| Integrated Devices Technolgy, Inc.
| IBIS Model Of 82P2816
| BB_416
[IBIS ver]	3.2
[File name]	82p2816.ibs
[File Rev]	1.0
[Date]		Aug. 15, 2005
[Source]	Integrated Devices Technolgy, Inc.
[Notes]   1. Temperatures: typ=25C, min=90C, max=-40C .
   2. simulator: hspice
   3. The IBIS models are validated with hspice models
[Disclaimer]	 Integrated Device Technology, Inc. ("IDT") hereby grants
		 the user of this IBIS model a non-exclusive, nontransferable
		 license to use this IBIS model under the following terms.
		 The user is granted this license only to use the IBIS model
		 and is not granted rights to sell, copy (except as needed to
		 run the IBIS model), rent, lease or sub-license the IBIS model
		 in whole or in part, or in modified form to anyone. The User
		 may modify the IBIS model to suit its specific applications,
		 but rights to derivative works and such modifications shall
		 belong to IDT. This IBIS model is provided on an AS IS" basis
		 and IDT makes absolutely no warranty with respect to the
		 information contained herein. IDT DISCLAIMS AND CUSTOMER WAIVES
		 ALL WARRANTIES, EXPRESS AND IMPLIED, INCLUDING WARRANTIES
		 OF MERCHANTABILITY AND FITNESS FOR A PARTICULAR PURPOSE. THE
		 ENTIRE RISK AS TO QUALITY AND PERFORMANCE IS WITH THE USER ACCORDINGLY,
		 IN NO EVENT SHALL IDT BE LIABLE FOR ANY DIRECT OR
		 INDIRECT DAMAGES, WHETHER IN CONTRACT OR TORT, INCLUDING ANY
		 LOST PROFITS OR OTHER INCIDENTAL, CONSEQUENTIAL, EXEMPLARY, OR
		 PUNITIVE DAMAGES ARISING OUT OF THE USE OR APPLICATION OF THE
		 IBIS model. Further, IDT reserves the right to make changes
		 without notice to
[Copyright]	Copyright 2005, Integrated Devices Technolgy, Inc.,
   All Rights Reserved.
|   Component 82P2816
[Component]	82P2816
[Manufacturer]	Integrated Devices Technolgy, Inc.
[Package]
| variable   typ   min   max
R_pkg   0.32   0.20   0.57
L_pkg   6.21nH   3.81nH   11.4nH
C_pkg   0.91pF   0.37pF   2.25pF
[Pin]  signal_name   model_name   R_pin   L_pin   C_pin
AE16   A0   PITSN   0.40   7.41nH   0.70pF
AF16   A1   PITSN   0.37   7.24nH   0.37pF
AE13   A10   PITSN   0.27   4.86nH   0.56pF
AD15   A2   PITSN   0.26   4.33nH   0.64pF
AE15   A3   PITSN   0.33   6.06nH   0.49pF
AF15   A4   PITSN   0.33   5.99nH   0.58pF
AC14   A5   PITSN   0.25   4.16nH   0.63pF
AD14   A6   PITSN   0.30   4.76nH   0.64pF
AE14   A7   PITSN   0.31   5.65nH   0.58pF
AF14   A8   PITSN   0.34   5.72nH   0.72pF
AD13   A9   PITSN   0.30   5.24nH   0.59pF
AD17   ALE_AS   PITSN   0.34   5.34nH   0.60pF
AE20   CLKA   PITSN   0.38   7.14nH   0.65pF
AF20   CLKB   PITSN   0.41   7.05nH   0.83pF
AD20   CLKE1   PTT04   0.38   6.28nH   1.00pF
AC21   CLKT1   PTT04   0.35   5.62nH   1.33pF
AD18   CSB   PITSN   0.30   5.34nH   0.64pF
AF13   D0   PBRT16N   0.36   6.83nH   0.59pF
AC12   D1   PBRT16N   0.26   3.95nH   0.69pF
AD12   D2   PBRT16N   0.30   5.18nH   0.69pF
AE12   D3   PBRT16N   0.35   5.72nH   0.75pF
AF12   D4   PBRT16N   0.37   6.72nH   0.56pF
AD11   D5   PBRT16N   0.29   5.28nH   0.81pF
AE11   D6   PBRT16N   0.34   6.09nH   0.63pF
AF11   D7   PBRT16N   0.36   6.25nH   0.80pF
AD9   GPIO0   PBRT04N   0.32   6.20nH   0.71pF
AC8   GPIO1   PBRT04N   0.43   8.75nH   0.82pF
AC17   IM   PITSU   0.45   7.78nH   0.67pF
AD16   INT_MOTB   PITSU   0.29   5.28nH   0.51pF
AF18   INTB   PTT12   0.42   7.96nH   0.48pF
AD19   LLOS   PTT04   0.50   10.21nH   0.77pF
AC19   LLOS0   PTT04   0.45   9.39nH   1.11pF
AE21   MCKSEL0   PITSN   0.40   7.45nH   0.54pF
AD21   MCKSEL1   PITSN   0.41   7.14nH   1.10pF
AD22   MCKSEL2   PITSN   0.57   11.40nH   0.94pF
AC22   MCKSEL3   PITSN   0.40   6.68nH   1.45pF
AF21   MCLK   PITSN   0.42   8.45nH   0.66pF
AF9   OE   PITSD   0.35   6.85nH   0.69pF
AC16   P_SB   PITSU   0.37   6.39nH   0.61pF
AF7   RCLK0   PTT04   0.42   7.34nH   0.69pF
AA2   RCLK1   PTT04   0.36   6.69nH   0.90pF
C20   RCLK10   PTT04   0.29   5.80nH   1.00pF
B18   RCLK11   PTT04   0.26   5.42nH   0.77pF
A16   RCLK12   PTT04   0.29   5.69nH   0.74pF
C15   RCLK13   PTT04   0.26   4.86nH   0.82pF
B13   RCLK14   PTT04   0.27   5.50nH   0.79pF
A11   RCLK15   PTT04   0.27   5.04nH   0.73pF
A9   RCLK16   PTT04   0.27   5.65nH   0.70pF
AC1   RCLK2   PTT04   0.43   8.54nH   0.80pF
AE3   RCLK3   PTT04   0.47   9.14nH   1.07pF
AE5   RCLK4   PTT04   0.45   8.69nH   0.83pF
AF24   RCLK5   PTT04   0.44   8.13nH   0.80pF
AC25   RCLK6   PTT04   0.42   7.70nH   0.92pF
AA26   RCLK7   PTT04   0.40   7.33nH   0.90pF
Y23   RCLK8   PTT04   0.28   6.52nH   1.24pF
B22   RCLK9   PTT04   0.34   7.73nH   0.94pF
AC6   RDN0   PTT04   0.35   5.67nH   1.41pF
AA1   RDN1   PTT04   0.38   8.17nH   0.95pF
D20   RDN10   PTT04   0.24   4.90nH   1.14pF
C18   RDN11   PTT04   0.26   5.24nH   0.78pF
B16   RDN12   PTT04   0.27   5.43nH   0.71pF
A14   RDN13   PTT04   0.31   5.99nH   0.73pF
C13   RDN14   PTT04   0.24   4.71nH   0.71pF
B11   RDN15   PTT04   0.26   4.90nH   0.76pF
B9   RDN16   PTT04   0.25   5.10nH   0.70pF
AB4   RDN2   PTT04   0.30   6.29nH   1.11pF
AF3   RDN3   PTT04   0.42   8.76nH   1.09pF
AF5   RDN4   PTT04   0.47   8.87nH   1.09pF
AD23   RDN5   PTT04   0.36   6.90nH   0.93pF
AC26   RDN6   PTT04   0.43   7.66nH   1.32pF
AB23   RDN7   PTT04   0.30   5.43nH   1.02pF
Y24   RDN8   PTT04   0.29   5.96nH   0.91pF
A21   RDN9   PTT04   0.33   6.98nH   0.73pF
AD6   RDP0   PTT04   0.50   9.80nH   0.86pF
Y4   RDP1   PTT04   0.30   5.75nH   0.84pF
A19   RDP10   PTT04   0.27   5.86nH   0.78pF
D18   RDP11   PTT04   0.25   4.86nH   0.75pF
C16   RDP12   PTT04   0.25   5.00nH   0.67pF
B14   RDP13   PTT04   0.28   5.78nH   0.76pF
A12   RDP14   PTT04   0.29   5.83nH   0.64pF
A10   RDP15   PTT04   0.28   5.49nH   0.70pF
C9   RDP16   PTT04   0.23   4.60nH   0.72pF
AB3   RDP2   PTT04   0.36   6.99nH   0.79pF
AD2   RDP3   PTT04   0.45   8.78nH   0.85pF
AD4   RDP4   PTT04   0.42   8.21nH   0.81pF
AE23   RDP5   PTT04   0.43   7.75nH   0.70pF
AD24   RDP6   PTT04   0.41   7.22nH   0.89pF
AB24   RDP7   PTT04   0.36   6.65nH   0.81pF
Y25   RDP8   PTT04   0.36   7.67nH   0.78pF
B21   RDP9   PTT04   0.27   5.92nH   0.91pF
A22   REF   NC   NA   NA   NA
AE19   REFA   PTT12   0.39   7.37nH   0.44pF
AF19   REFB   PTT12   0.40   7.92nH   0.93pF
AE9   RIM   PITSD   0.36   6.95nH   0.50pF
J4   RRING0   NC   0.32   5.12nH   1.05pF
L3   RRING1   NC   0.31   6.06nH   1.01pF
G23   RRING10   NC   0.32   5.29nH   0.96pF
E24   RRING11   NC   0.32   5.38nH   0.98pF
C23   RRING12   NC   0.30   5.54nH   1.00pF
D6   RRING13   NC   0.26   4.98nH   1.05pF
C4   RRING14   NC   0.38   6.31nH   1.24pF
E4   RRING15   NC   0.39   6.64nH   1.12pF
G3   RRING16   NC   0.36   6.02nH   1.03pF
N4   RRING2   NC   0.29   4.54nH   1.29pF
R3   RRING3   NC   0.27   4.73nH   0.89pF
U4   RRING4   NC   0.26   4.42nH   0.96pF
U24   RRING5   NC   0.26   4.49nH   0.93pF
R23   RRING6   NC   0.26   4.72nH   0.94pF
N24   RRING7   NC   0.29   5.10nH   0.97pF
L23   RRING8   NC   0.31   5.38nH   1.01pF
J24   RRING9   NC   0.32   5.56nH   0.94pF
AF10   RSTB   PITSU   0.35   6.73nH   0.53pF
K4   RTIP0   NC   0.31   4.78nH   0.99pF
M3   RTIP1   NC   0.31   5.32nH   0.89pF
H23   RTIP10   NC   0.31   4.90nH   1.01pF
F24   RTIP11   NC   0.31   5.06nH   1.01pF
C24   RTIP12   NC   0.33   5.93nH   0.98pF
D5   RTIP13   NC   0.29   5.65nH   1.09pF
C3   RTIP14   NC   0.43   7.34nH   1.28pF
F4   RTIP15   NC   0.37   5.90nH   1.11pF
H3   RTIP16   NC   0.36   5.69nH   1.02pF
P4   RTIP2   NC   0.29   4.22nH   0.90pF
T3   RTIP3   NC   0.28   4.73nH   0.90pF
V4   RTIP4   NC   0.25   4.43nH   0.96pF
V24   RTIP5   NC   0.28   4.39nH   0.86pF
T23   RTIP6   NC   0.26   4.38nH   0.87pF
P24   RTIP7   NC   0.28   4.81nH   0.94pF
M23   RTIP8   NC   0.30   4.99nH   0.94pF
K24   RTIP9   NC   0.33   5.27nH   0.91pF
AE18   SCLK_DSB_RDB PITSN   0.38   7.33nH   0.44pF
AF17   SDI_RWB_WRB  PITSN   0.36   6.18nH   0.81pF
AE17   SDO_RDY_ACKB PTT12   0.37   6.87nH   0.50pF
AE8   TCK   PITSN   0.34   6.60nH   0.79pF
AE6   TCLK0   PITSN   0.36   6.58nH   0.95pF
Y3   TCLK1   PITSN   0.30   6.37nH   0.93pF
B19   TCLK10   PITSN   0.27   5.54nH   0.71pF
A17   TCLK11   PITSN   0.28   5.61nH   0.59pF
D16   TCLK12   PITSN   0.23   4.59nH   0.68pF
C14   TCLK13   PITSN   0.26   5.21nH   0.76pF
B12   TCLK14   PITSN   0.27   5.22nH   0.67pF
B10   TCLK15   PITSN   0.26   4.92nH   0.69pF
A8   TCLK16   PITSN   0.28   5.85nH   0.74pF
AB2   TCLK2   PITSN   0.36   7.82nH   1.15pF
AD1   TCLK3   PITSN   0.40   8.44nH   1.06pF
AE4   TCLK4   PITSN   0.41   8.03nH   1.00pF
AF23   TCLK5   PITSN   0.44   8.36nH   0.92pF
AD25   TCLK6   PITSN   0.38   7.14nH   1.06pF
AB25   TCLK7   PITSN   0.41   7.68nH   0.72pF
Y26   TCLK8   PITSN   0.35   7.15nH   1.00pF
C21   TCLK9   PITSN   0.26   5.51nH   0.98pF
AF8   TDI   PITSU   0.41   8.18nH   0.52pF
AF6   TDN0   PBRT04N   0.43   8.17nH   0.73pF
Y2   TDN1   PBRT04N   0.35   6.90nH   0.92pF
C19   TDN10   PBRT04N   0.25   4.99nH   0.81pF
B17   TDN11   PBRT04N   0.26   5.14nH   0.70pF
A15   TDN12   PBRT04N   0.29   5.51nH   0.78pF
D14   TDN13   PBRT04N   0.22   4.56nH   0.79pF
C12   TDN14   PBRT04N   0.24   4.72nH   0.70pF
C10   TDN15   PBRT04N   0.23   4.41nH   0.71pF
B8   TDN16   PBRT04N   0.25   5.28nH   0.84pF
AB1   TDN2   PBRT04N   0.41   8.52nH   0.90pF
AC3   TDN3   PBRT04N   0.41   7.58nH   0.89pF
AF4   TDN4   PBRT04N   0.49   9.85nH   0.79pF
AE22   TDN5   PBRT04N   0.41   7.56nH   0.65pF
AD26   TDN6   PBRT04N   0.46   8.78nH   0.86pF
AB26   TDN7   PBRT04N   0.44   7.97nH   0.78pF
AA24   TDN8   PBRT04N   0.35   6.61nH   0.76pF
A20   TDN9   PBRT04N   0.33   6.61nH   0.84pF
AD8   TDO   PTT12   0.38   6.77nH   0.91pF
AD5   TDP0   PITSN   0.42   7.76nH   0.81pF
Y1   TDP1   PITSN   0.34   7.19nH   0.79pF
A18   TDP10   PITSN   0.32   6.80nH   0.84pF
C17   TDP11   PITSN   0.24   4.67nH   0.79pF
B15   TDP12   PITSN   0.26   5.17nH   0.79pF
A13   TDP13   PITSN   0.28   5.83nH   0.77pF
D12   TDP14   PITSN   0.22   4.12nH   0.77pF
D10   TDP15   PITSN   0.20   3.81nH   0.79pF
C8   TDP16   PITSN   0.22   4.88nH   0.97pF
AA3   TDP2   PITSN   0.31   6.44nH   1.06pF
AC2   TDP3   PITSN   0.42   8.09nH   0.96pF
AD3   TDP4   PITSN   0.44   8.65nH   1.20pF
AF22   TDP5   PITSN   0.44   7.92nH   0.65pF
AE24   TDP6   PITSN   0.43   8.64nH   1.31pF
AC24   TDP7   PITSN   0.33   6.40nH   1.09pF
AA25   TDP8   PITSN   0.31   6.32nH   1.03pF
B20   TDP9   PITSN   0.35   8.02nH   1.08pF
AC10   TEHW   PITSU   0.31   5.51nH   0.92pF
AD10   TEHWE   PITSU   0.31   6.26nH   0.81pF
AE10   TESTSE   PITSD   0.31   5.75nH   0.87pF
AD7   TMS   PITSU   0.45   7.74nH   1.63pF
J1   TRING0   NC   0.29   5.90nH   0.97pF
L1   TRING1   NC   0.29   5.30nH   0.95pF
G26   TRING10   NC   0.29   5.39nH   1.02pF
E26   TRING11   NC   0.30   5.94nH   1.08pF
A23   TRING12   NC   0.32   6.88nH   1.09pF
A6   TRING13   NC   0.31   7.09nH   1.09pF
A4   TRING14   NC   0.40   7.45nH   1.28pF
E1   TRING15   NC   0.32   6.01nH   1.11pF
G1   TRING16   NC   0.32   6.06nH   1.14pF
N1   TRING2   NC   0.25   5.65nH   0.98pF
R1   TRING3   NC   0.27   5.94nH   0.88pF
U1   TRING4   NC   0.28   6.79nH   0.96pF
U26   TRING5   NC   0.25   5.69nH   0.96pF
R26   TRING6   NC   0.26   5.20nH   0.96pF
N26   TRING7   NC   0.27   5.72nH   0.95pF
L26   TRING8   NC   0.27   5.47nH   0.96pF
J26   TRING9   NC   0.29   5.66nH   1.04pF
AE7   TRSTB   PITSD   0.38   7.02nH   0.72pF
K1   TTIP0   NC   0.29   6.28nH   0.71pF
M1   TTIP1   NC   0.30   5.62nH   0.86pF
H26   TTIP10   NC   0.30   5.18nH   0.86pF
F26   TTIP11   NC   0.30   5.88nH   0.88pF
A24   TTIP12   NC   0.33   6.81nH   1.02pF
A5   TTIP13   NC   0.31   6.92nH   1.00pF
A3   TTIP14   NC   0.39   7.47nH   1.25pF
F1   TTIP15   NC   0.32   5.67nH   0.95pF
H1   TTIP16   NC   0.32   6.37nH   0.91pF
P1   TTIP2   NC   0.25   5.00nH   0.80pF
T1   TTIP3   NC   0.26   6.10nH   0.81pF
V1   TTIP4   NC   0.28   6.92nH   0.78pF
V26   TTIP5   NC   0.24   5.77nH   0.83pF
T26   TTIP6   NC   0.24   5.49nH   0.75pF
P26   TTIP7   NC   0.25   5.33nH   0.75pF
M26   TTIP8   NC   0.27   5.79nH   0.83pF
K26   TTIP9   NC   0.28   5.47nH   0.83pF
W3   VCOM0   NC   NA   NA   NA
W24   VCOM1   NC   NA   NA   NA
W4   VCOMEN   NC   NA   NA   NA
J3   VDDR0   POWER   0.30   5.86nH   0.94pF
K3   VDDR1   POWER   0.31   5.81nH   1.00pF
G24   VDDR10   POWER   0.33   5.15nH   1.54pF
D24   VDDR11   POWER   0.30   5.93nH   1.07pF
D23   VDDR12   POWER   0.25   5.14nH   1.01pF
C6   VDDR13   POWER   0.29   5.22nH   1.42pF
C5   VDDR14   POWER   0.34   5.74nH   1.33pF
E3   VDDR15   POWER   0.38   6.27nH   2.00pF
F3   VDDR16   POWER   0.34   6.64nH   1.14pF
N3   VDDR2   POWER   0.32   5.37nH   0.92pF
P3   VDDR3   POWER   0.26   5.47nH   0.88pF
U3   VDDR4   POWER   0.25   4.54nH   0.93pF
T24   VDDR5   POWER   0.26   4.56nH   1.00pF
R24   VDDR6   POWER   0.26   5.39nH   0.96pF
M24   VDDR7   POWER   0.27   5.57nH   0.96pF
L24   VDDR8   POWER   0.32   6.62nH   1.10pF
H24   VDDR9   POWER   0.31   6.19nH   0.96pF
J2   VDDT0   POWER   0.28   5.79nH   1.19pF
K2   VDDT1   POWER   0.27   5.23nH   1.14pF
G25   VDDT10   POWER   0.28   5.38nH   1.13pF
B24   VDDT11   POWER   0.34   7.03nH   1.64pF
B23   VDDT12   POWER   0.28   5.70nH   1.38pF
B6   VDDT13   POWER   0.29   6.24nH   1.61pF
B5   VDDT14   POWER   0.32   7.07nH   2.25pF
E2   VDDT15   POWER   0.32   5.69nH   1.40pF
F2   VDDT16   POWER   0.29   6.03nH   1.16pF
N2   VDDT2   POWER   0.25   5.17nH   1.12pF
P2   VDDT3   POWER   0.27   5.85nH   1.19pF
U2   VDDT4   POWER   0.24   6.43nH   1.43pF
T25   VDDT5   POWER   0.24   5.89nH   1.16pF
R25   VDDT6   POWER   0.22   4.62nH   1.10pF
M25   VDDT7   POWER   0.24   4.97nH   1.22pF
L25   VDDT8   POWER   0.25   5.23nH   1.15pF
H25   VDDT9   POWER   0.27   5.41nH   1.16pF
K10   GNDD   GND   NA   NA   NA
K11   GNDD   GND   NA   NA   NA
K12   GNDD   GND   NA   NA   NA
K13   GNDD   GND   NA   NA   NA
K14   GNDD   GND   NA   NA   NA
K15   GNDD   GND   NA   NA   NA
K16   GNDD   GND   NA   NA   NA
K17   GNDD   GND   NA   NA   NA
L10   GNDD   GND   NA   NA   NA
L11   GNDD   GND   NA   NA   NA
L12   GNDD   GND   NA   NA   NA
L13   GNDD   GND   NA   NA   NA
L14   GNDD   GND   NA   NA   NA
L15   GNDD   GND   NA   NA   NA
L16   GNDD   GND   NA   NA   NA
L17   GNDD   GND   NA   NA   NA
M10   GNDD   GND   NA   NA   NA
M11   GNDD   GND   NA   NA   NA
M12   GNDD   GND   NA   NA   NA
M13   GNDD   GND   NA   NA   NA
M14   GNDD   GND   NA   NA   NA
M15   GNDD   GND   NA   NA   NA
M16   GNDD   GND   NA   NA   NA
M17   GNDD   GND   NA   NA   NA
N10   GNDD   GND   NA   NA   NA
N11   GNDD   GND   NA   NA   NA
N12   GNDD   GND   NA   NA   NA
N13   GNDD   GND   NA   NA   NA
N14   GNDD   GND   NA   NA   NA
N15   GNDD   GND   NA   NA   NA
N16   GNDD   GND   NA   NA   NA
N17   GNDD   GND   NA   NA   NA
P10   GNDD   GND   NA   NA   NA
P11   GNDD   GND   NA   NA   NA
P12   GNDD   GND   NA   NA   NA
P13   GNDD   GND   NA   NA   NA
P14   GNDD   GND   NA   NA   NA
P15   GNDD   GND   NA   NA   NA
P16   GNDD   GND   NA   NA   NA
P17   GNDD   GND   NA   NA   NA
R10   GNDD   GND   NA   NA   NA
R11   GNDD   GND   NA   NA   NA
R12   GNDD   GND   NA   NA   NA
R13   GNDD   GND   NA   NA   NA
R14   GNDD   GND   NA   NA   NA
R15   GNDD   GND   NA   NA   NA
R16   GNDD   GND   NA   NA   NA
R17   GNDD   GND   NA   NA   NA
T10   GNDD   GND   NA   NA   NA
T11   GNDD   GND   NA   NA   NA
T12   GNDD   GND   NA   NA   NA
T13   GNDD   GND   NA   NA   NA
T14   GNDD   GND   NA   NA   NA
T15   GNDD   GND   NA   NA   NA
T16   GNDD   GND   NA   NA   NA
T17   GNDD   GND   NA   NA   NA
U10   GNDD   GND   NA   NA   NA
U11   GNDD   GND   NA   NA   NA
U12   GNDD   GND   NA   NA   NA
U13   GNDD   GND   NA   NA   NA
U14   GNDD   GND   NA   NA   NA
U15   GNDD   GND   NA   NA   NA
U16   GNDD   GND   NA   NA   NA
U17   GNDD   GND   NA   NA   NA
A1   GNDA   GND   NA   NA   NA
A2   GNDA   GND   NA   NA   NA
A25   GNDA   GND   NA   NA   NA
A26   GNDA   GND   NA   NA   NA
B1   GNDA   GND   NA   NA   NA
B2   GNDA   GND   NA   NA   NA
B25   GNDA   GND   NA   NA   NA
B26   GNDA   GND   NA   NA   NA
D4   GNDA   GND   NA   NA   NA
E23   GNDA   GND   NA   NA   NA
F23   GNDA   GND   NA   NA   NA
G4   GNDA   GND   NA   NA   NA
H4   GNDA   GND   NA   NA   NA
J23   GNDA   GND   NA   NA   NA
K23   GNDA   GND   NA   NA   NA
L4   GNDA   GND   NA   NA   NA
M4   GNDA   GND   NA   NA   NA
N23   GNDA   GND   NA   NA   NA
P23   GNDA   GND   NA   NA   NA
R4   GNDA   GND   NA   NA   NA
T4   GNDA   GND   NA   NA   NA
U23   GNDA   GND   NA   NA   NA
V23   GNDA   GND   NA   NA   NA
V2   GNDA   GND   NA   NA   NA
V3   GNDA   GND   NA   NA   NA
AE1   GNDA   GND   NA   NA   NA
AE2   GNDA   GND   NA   NA   NA
AE25   GNDA   GND   NA   NA   NA
AE26   GNDA   GND   NA   NA   NA
AF1   GNDA   GND   NA   NA   NA
AF2   GNDA   GND   NA   NA   NA
AF25   GNDA   GND   NA   NA   NA
AF26   GNDA   GND   NA   NA   NA
B3   GNDT   GND   NA   NA   NA
B4   GNDT   GND   NA   NA   NA
D3   GNDT   GND   NA   NA   NA
E25   GNDT   GND   NA   NA   NA
F25   GNDT   GND   NA   NA   NA
G2   GNDT   GND   NA   NA   NA
H2   GNDT   GND   NA   NA   NA
J25   GNDT   GND   NA   NA   NA
K25   GNDT   GND   NA   NA   NA
L2   GNDT   GND   NA   NA   NA
M2   GNDT   GND   NA   NA   NA
N25   GNDT   GND   NA   NA   NA
P25   GNDT   GND   NA   NA   NA
R2   GNDT   GND   NA   NA   NA
T2   GNDT   GND   NA   NA   NA
U25   GNDT   GND   NA   NA   NA
V25   GNDT   GND   NA   NA   NA
C1   VDDA   POWER   NA   NA   NA
C2   VDDA   POWER   NA   NA   NA
C25   VDDA   POWER   NA   NA   NA
C26   VDDA   POWER   NA   NA   NA
D1   VDDA   POWER   NA   NA   NA
D2   VDDA   POWER   NA   NA   NA
D25   VDDA   POWER   NA   NA   NA
D26   VDDA   POWER   NA   NA   NA
W1   VDDA   POWER   NA   NA   NA
W2   VDDA   POWER   NA   NA   NA
W25   VDDA   POWER   NA   NA   NA
W26   VDDA   POWER   NA   NA   NA
A7   VDDIO   POWER   NA   NA   NA
B7   VDDIO   POWER   NA   NA   NA
C7   VDDIO   POWER   NA   NA   NA
D7   VDDIO   POWER   NA   NA   NA
D8   VDDIO   POWER   NA   NA   NA
D9   VDDIO   POWER   NA   NA   NA
D19   VDDIO   POWER   NA   NA   NA
D21   VDDIO   POWER   NA   NA   NA
D22   VDDIO   POWER   NA   NA   NA
W23   VDDIO   POWER   NA   NA   NA
AA4   VDDIO   POWER   NA   NA   NA
AA23   VDDIO   POWER   NA   NA   NA
AC4   VDDIO   POWER   NA   NA   NA
AC11   VDDIO   POWER   NA   NA   NA
AC13   VDDIO   POWER   NA   NA   NA
AC15   VDDIO   POWER   NA   NA   NA
C11   VDDD   POWER   NA   NA   NA
D11   VDDD   POWER   NA   NA   NA
D13   VDDD   POWER   NA   NA   NA
D15   VDDD   POWER   NA   NA   NA
D17   VDDD   POWER   NA   NA   NA
AC5   VDDD   POWER   NA   NA   NA
AC7   VDDD   POWER   NA   NA   NA
AC9   VDDD   POWER   NA   NA   NA
AC18   VDDD   POWER   NA   NA   NA
AC20   VDDD   POWER   NA   NA   NA
AC23   VDDD   POWER   NA   NA   NA
C22   NC   NC   NA   NA   NA
| Models and submodels in the file (7): PBRT04N (I/O), PBRT16N (I/O), PITSD (Input), PITSN (Input), PITSU (Input), PTT04 (3-state), PTT12 (3-state)
